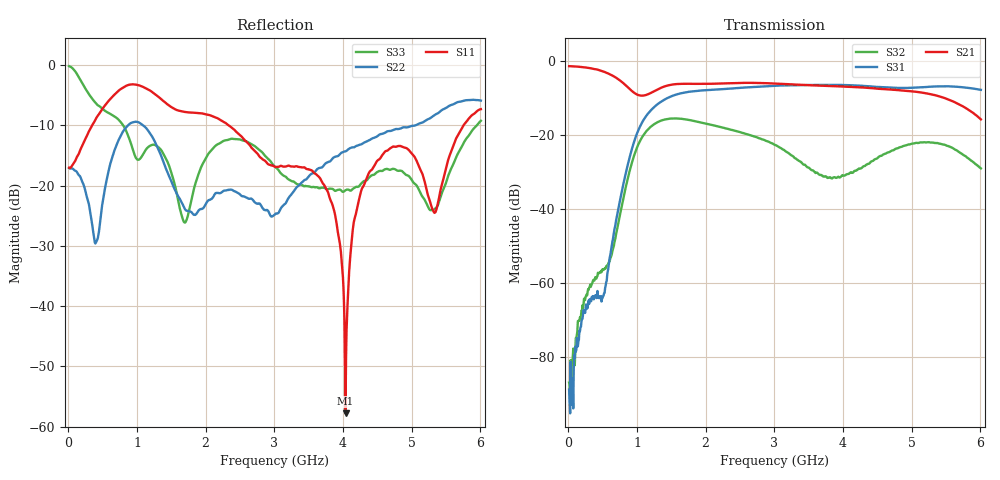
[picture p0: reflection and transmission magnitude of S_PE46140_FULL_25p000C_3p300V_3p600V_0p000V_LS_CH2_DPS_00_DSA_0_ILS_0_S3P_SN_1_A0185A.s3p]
! Device ID: PE46140_FULL
! File Path: z:\PE46140\MajorStates\25p000C\3p300\LS_CH2_DPS_00_DSA_0_ILS_0\PE46140_FULL_25p000C_3p300V_3p600V_0p000V_LS_CH2_DPS_00_DSA_0_ILS_0_S3P_SN_1_A0185A.s3p
! Serial: 1
! Lot: A0185A
! Temp: 25.000C
! VDD: 3.300
! VSS: 0.000
! Control_Hi: 3.600
! Control_Lo: 0.000
! Logic State: LS_CH2_DPS_00_DSA_0_ILS_0
! Port 1: RFIN
! Port 2: RFOUT1
! Port 3: RFOUT2
! ThroughPath:1-3
! IDD: 0.0003148417
! ISS: -9.22e-008
! Comment:
#  Hz  S  RI  R  50
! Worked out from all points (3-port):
!   801 points, 10 MHz to 6.01 GHz, reference 50 ohm
!   strongest paths, dB at 10 MHz, 1.51 GHz, 3.01 GHz, 4.51 GHz, 6.01 GHz:
!     S21: -1.5, -6.5, -6.2, -7.6, -15.8
!     S31: -88.7, -9.5, -6.8, -7.1, -7.9
!     S32: -86.8, -15.6, -22.7, -26.1, -29.1
!   lowest |S11| = -57.8 dB at 4.037 GHz (marker M1), VSWR 1.00, Z = 49.9 + j0.0424 ohm
!   |S11| at or under -10 dB: start of sweep to 346.2 MHz; 2.333 GHz to 5.756 GHz (3.424 GHz wide, 84.6 % of centre)
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1e7  0.1401 -0.0109  0.8421 -0.0246  -4.46e-05 -1.2e-05
     0.8417 -0.0242  0.14 -0.00676  -3.29e-05 5.02e-05
     -1.59e-05 3.29e-05  7.21e-07 -4.55e-05  0.9747 -0.0928
3.55e8  -0.0161 -0.3218  0.4592 -0.6282  -0.000559 -0.000312
        0.4592 -0.6262  -0.00909 -0.0426  -0.000178 0.00107
        -0.000577 -0.000336  -0.000115 0.00105  -0.4602 -0.2357
1.165e9  -0.5853 0.2238  -0.2048 -0.2878  -0.1934 -0.0289
         -0.205 -0.2885  0.2134 -0.1871  -0.00286 0.1196
         -0.1936 -0.0293  -0.00314 0.1197  0.1752 0.1143
1.9825e9  -0.1843 0.3467  -0.418 0.2478  0.3938 -0.0581
          -0.4182 0.2475  0.0622 -0.0259  -0.1419 -0.0176
          0.3941 -0.0581  -0.1419 -0.0178  0.0449 0.1549
3.01e9  0.018 0.1418  0.4092 0.2718  -0.3949 -0.2327
        0.4089 0.2726  -0.0576 -0.00135  0.0653 -0.0322
        -0.3952 -0.233  0.0653 -0.0323  0.1336 -0.0511
3.7675e9  0.0256 0.0881  0.2754 -0.3639  -0.247 0.4012
          0.2759 -0.3637  0.0773 0.1345  -0.0149 0.0218
          -0.2472 0.4009  -0.015 0.0218  0.0896 -0.022
4.0375e9  -0.00122 0.000425  0.0428 -0.4428  -0.00934 0.4684
          0.0431 -0.4433  0.1395 0.1324  0.0241 0.0157
          -0.00881 0.4678  0.0239 0.0155  0.0882 -0.0243
4.3825e9  -0.103 -0.0771  -0.2531 -0.3447  0.2699 0.3609
          -0.2531 -0.3453  0.2158 0.0992  0.0157 -0.0378
          0.2702 0.3603  0.0156 -0.0378  0.1111 -0.0364
5.335e9  -0.0418 -0.042  -0.1082 0.3253  0.3313 -0.3017
         -0.1091 0.3253  0.3832 -0.0379  0.0115 0.0769
         0.3318 -0.301  0.0113 0.0768  0.0635 0.0043
6.01e9  -0.2951 -0.3133  0.1535 0.0484  -0.2001 -0.349
        0.1539 0.0486  0.2469 -0.4427  0.0295 -0.0187
        -0.2017 -0.3499  0.0297 -0.019  0.3152 0.14
